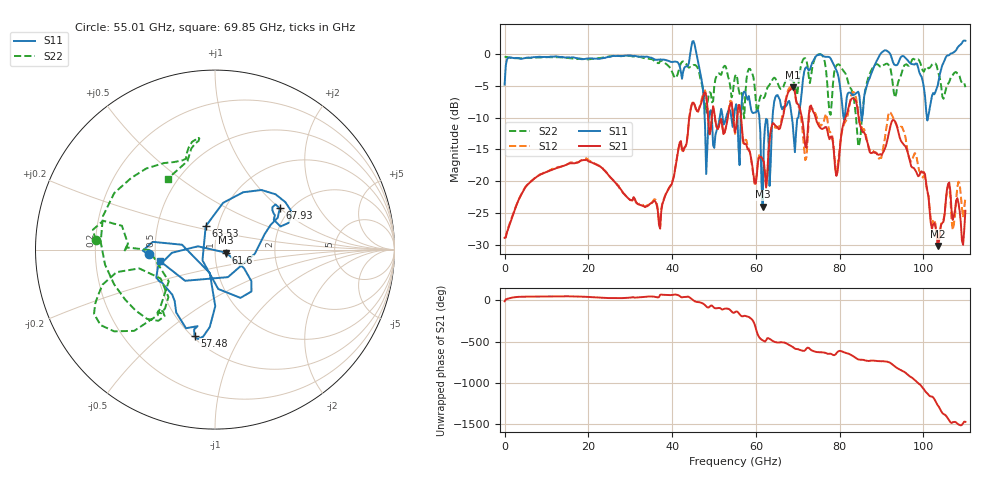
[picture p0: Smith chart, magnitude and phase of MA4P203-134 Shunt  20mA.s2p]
!Keysight Technologies,N5247B,US61255204,A.15.70.20
!Date: Friday, October 21, 2022 15:23:32
!Correction: S11(C  4-Port  )
!S31(C  4-Port  )
!S13(C  4-Port  )
!S33(C  4-Port  )
!S2P File: Measurements: S11, S31, S13, S33:
# Hz S  dB  R 50
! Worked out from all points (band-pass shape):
!   401 points, 10 MHz to 110 GHz, reference 50 ohm
!   highest |S21| = -5.21 dB at 68.75 GHz (marker M1); lowest = -30.1 dB at 103.4 GHz (marker M2)
!   |S21| within 3 dB of the highest: 66.92 GHz to 70.33 GHz (3.414 GHz wide, 4.98 % of centre); 82.19 GHz to 84.15 GHz (1.96 GHz wide, 2.36 % of centre)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
!   lowest |S11| = -24.0 dB at 61.6 GHz (marker M3), VSWR 1.14, Z = 56.5 - j1.93 ohm
!   |S11| at or under -10 dB: 49.44 GHz to 51.36 GHz (1.913 GHz wide, 3.8 % of centre); 60.82 GHz to 63.97 GHz (3.15 GHz wide, 5.05 % of centre); 68.59 GHz to 70.09 GHz (1.501 GHz wide, 2.17 % of centre)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
!   |S22| runs from -14.5 to 0.0 dB; largest |S21 - S12| = 0.17
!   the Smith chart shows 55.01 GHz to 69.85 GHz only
!   S11 on the Smith chart (normalised r, x): 55.01 GHz: 0.46, -0.03; 57.48 GHz: 0.51, -0.65; 61.6 GHz: 1.13, -0.04; 63.53 GHz: 0.87, +0.23; 67.93 GHz: 1.77, +1.00; 69.85 GHz: 0.53, -0.08
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1e7  -4.81 -179.7  -28.87 -9.7  -28.89 -9.8  -0.49 -179.7
1.843332e10  -0.83 145.7  -16.70 46.7  -16.68 46.6  -0.77 145.3
3.685665e10  -0.90 154.6  -26.79 40.1  -26.39 40.6  -1.44 154.3
4.51059e10  2.02 85.1  -7.65 -0.3  -7.61 -2.5  -1.75 115.3
4.813062e10  -18.85 60.1  -6.58 -71.5  -6.41 -71.9  -9.23 113.3
5.5005e10  -8.62 -175.8  -12.29 -142.6  -12.54 -144.1  -3.52 175.6
5.747978e10  -6.12 -103.3  -14.09 172.8  -13.46 178.1  -6.27 -131.1
6.16044e10  -23.96 -15.6  -16.55 -122.8  -16.66 -120.7  -6.74 -132.9
6.352922e10  -17.08 111.7  -12.04 -113.5  -12.41 -110.3  -4.51 -161.1
6.792882e10  -7.37 32.5  -5.79 -179.2  -5.38 179.5  -4.08 99.0
6.875375e10  -10.81 17.0  -5.21 157.9  -4.94 154.0  -4.26 98.6
6.985365e10  -10.14 -167.7  -7.82 131.2  -8.10 130.9  -6.47 123.5
7.342832e10  -1.38 178.3  -8.68 112.2  -8.66 107.6  -2.24 156.3
7.645305e10  -0.44 -165.6  -11.52 87.1  -9.92 118.9  -1.30 148.0
7.947778e10  -3.01 -147.5  -18.57 96.4  -17.77 95.0  -1.65 -137.2
8.415235e10  -6.05 -39.1  -8.22 12.9  -7.75 17.9  -12.29 -170.3
8.745205e10  -3.22 49.8  -15.58 -8.4  -15.22 5.2  -2.70 53.6
9.185165e10  0.20 88.6  -12.06 -30.5  -9.09 -22.9  -1.92 76.1
9.817608e10  -1.48 176.0  -18.41 105.0  -15.72 104.0  -0.95 -174.5
1.034006e11  -4.93 -37.5  -30.13 169.9  -30.18 173.7  -2.59 -110.9
1.069753e11  0.16 10.4  -26.06 -34.1  -27.64 -37.2  -3.31 -23.4
1.1e11  2.07 46.1  -24.62 -29.7  -22.60 -27.4  -5.22 10.5
